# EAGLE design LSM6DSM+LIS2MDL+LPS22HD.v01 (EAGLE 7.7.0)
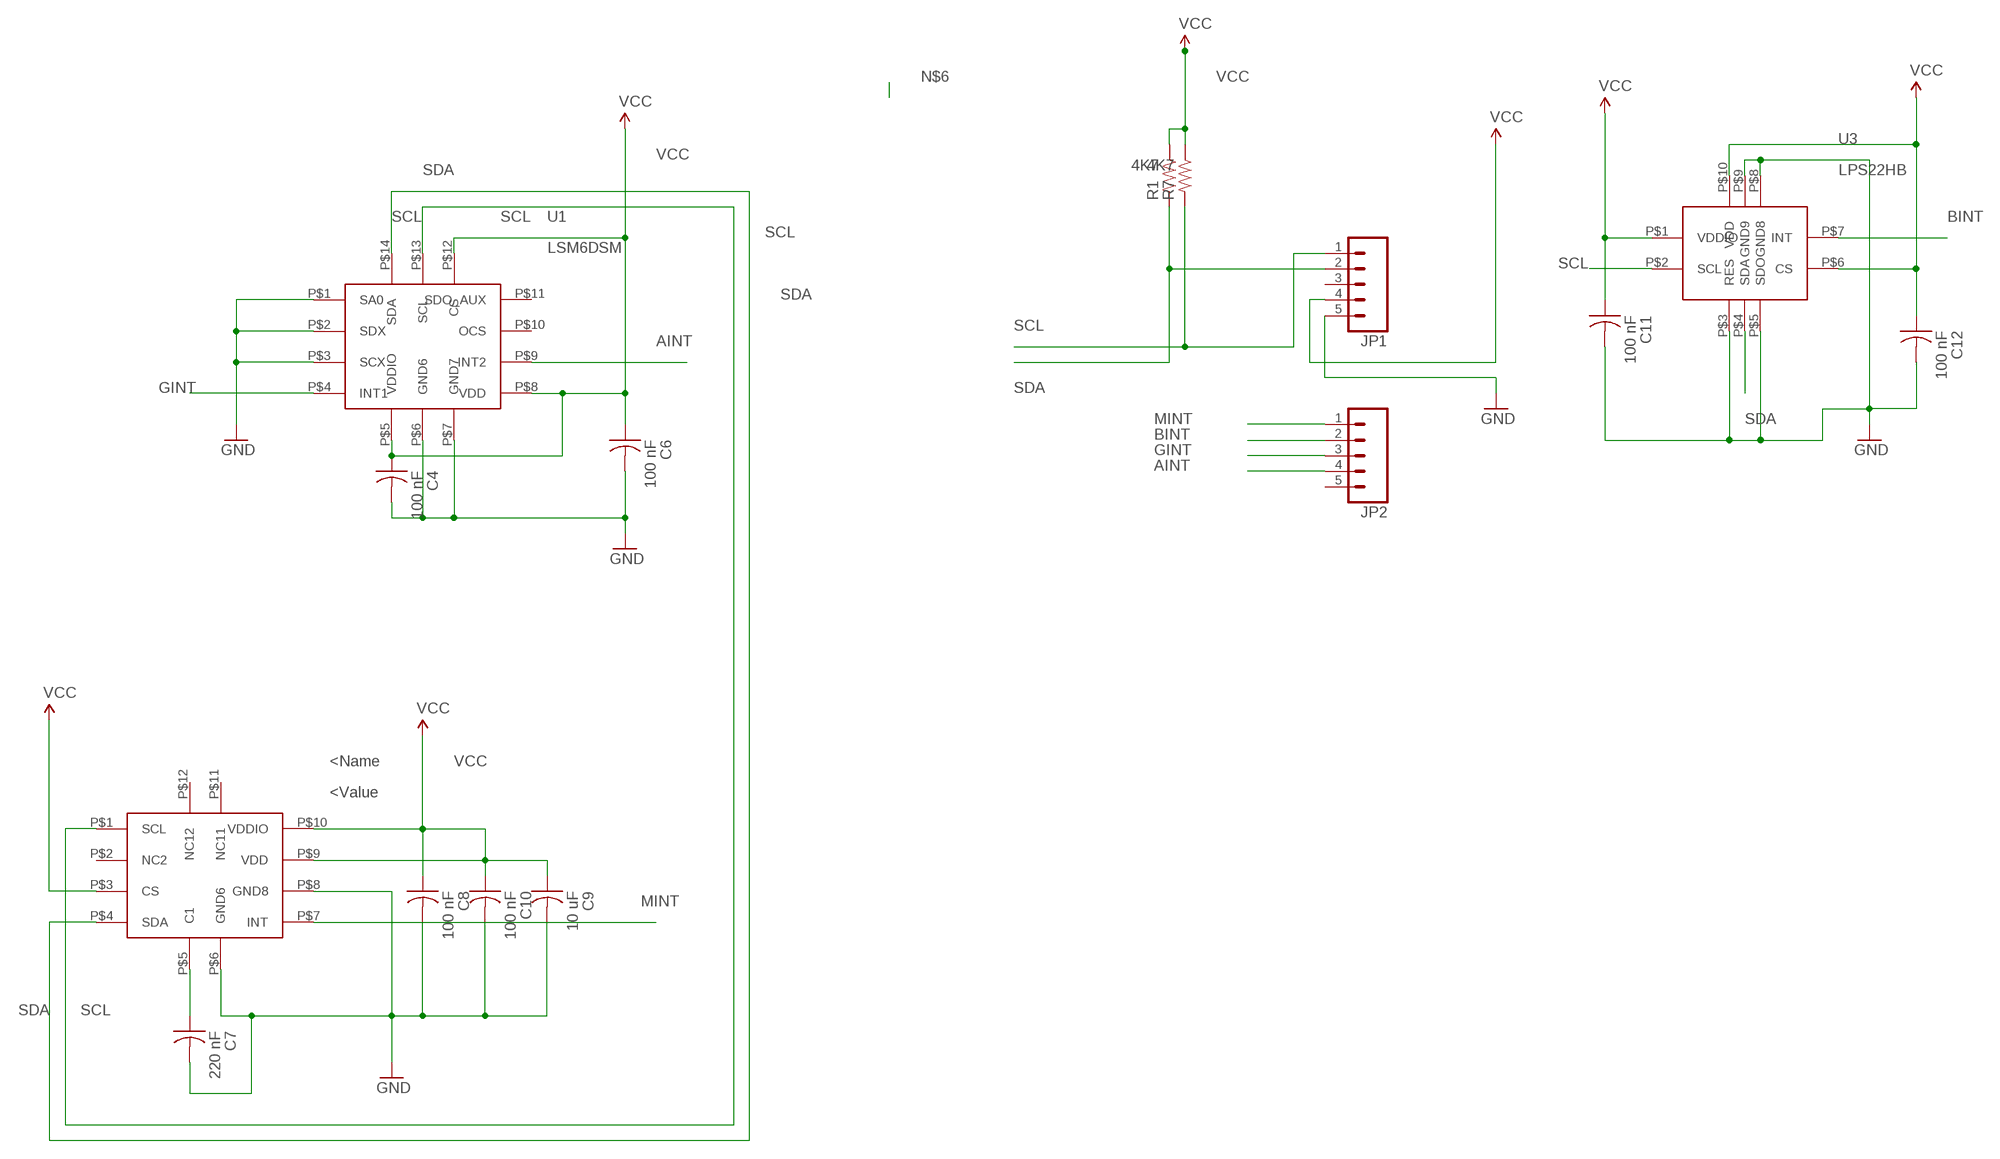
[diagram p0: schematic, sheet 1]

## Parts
C4  100 nF  C-US  [C0402_B]
C6  100 nF  C-US  [C0402_B]
C7  220 nF  C-US  [C0402_B]
C8  100 nF  C-US  [C0402_B]
C9  10 uF  C-US  [C0402_B]
C10  100 nF  C-US  [C0402_B]
C11  100 nF  C-US  [C0402_B]
C12  100 nF  C-US  [C0402_B]
JP1  M05NO_SILK  [1X05_NO_SILK]
JP2  M05NO_SILK  [1X05_NO_SILK]
R1  4K7  R-US_  [R0402_B]
R7  4K7  R-US_  [R0402_B]
U1  LSM6DSM  [LSM6DSM]
U2  LIS2MDL  [LIS2MDL]
U3  LPS22HB  [LPS22HB]

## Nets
AINT: JP2.4 U1.P$9(INT2)
BINT: JP2.2 U3.P$7(INT)
GINT: JP2.3 U1.P$4(INT1)
GND: C4.2 C6.2 C7.2 C8.2 C9.2 C10.2 C11.2 C12.2 JP1.5 U1.P$1(SA0) U1.P$2(SDX) U1.P$3(SCX) U1.P$6(GND6) U1.P$7(GND7) U2.P$6(GND6) U2.P$8(GND8) U3.P$3(RES) U3.P$5(SDO) U3.P$8(GND8) U3.P$9(GND9)
MINT: JP2.1 U2.P$7(INT)
N$4: C7.1 U2.P$5(C1)
SCL: JP1.1 R7.2 U1.P$13(SCL) U2.P$1(SCL) U3.P$2(SCL)
SDA: JP1.2 R1.2 U1.P$14(SDA) U2.P$4(SDA) U3.P$4(SDA)
VCC: C4.1 C6.1 C8.1 C9.1 C10.1 C11.1 C12.1 JP1.4 R1.1 R7.1 U1.P$5(VDDIO) U1.P$8(VDD) U1.P$12(CS) U2.P$3(CS) U2.P$9(VDD) U2.P$10(VDDIO) U3.P$1(VDDIO) U3.P$6(CS) U3.P$10(VDD)
Unconnected: JP1.3 JP2.5 U2.P$2(NC2) U2.P$11(NC11) U2.P$12(NC12)

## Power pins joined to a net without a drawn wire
OCS: U1.P$10(OCS)
SDO_AUX: U1.P$11(SDO_AUX)

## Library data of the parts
C4 C6-C12 = Spark:C-US: Capacitor
JP1 JP2 = SparkFun-Connectors:M05: Header 5 Standard 5-pin 0.1" header. Use with straight break away headers (SKU : PRT-00116), right angle break away headers (PRT-00553), swiss pins (PRT-00743), machine pins (PRT-00117), and female headers (PRT-00115). Molex polarized connector foot print use with SKU : PRT-08230 with associated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
R1 R7 = Spark:R-US_: 0402 Resistor
U1 = Kris:LSM6DSM: LSM6DSM ST accel/gyro
U2 = Kris:LIS2MDL: LIS2MDL ST magnetomneter
U3 = Kris:LPS22HB: LPS22HB ST pressure sensor http://www.st.com/content/ccc/resource/technical/document/datasheet/bf/c1/4f/23/61/17/44/8a/DM00140895.pdf/files/DM00140895.pdf/jcr:content/translations/en.DM00140895.pdf

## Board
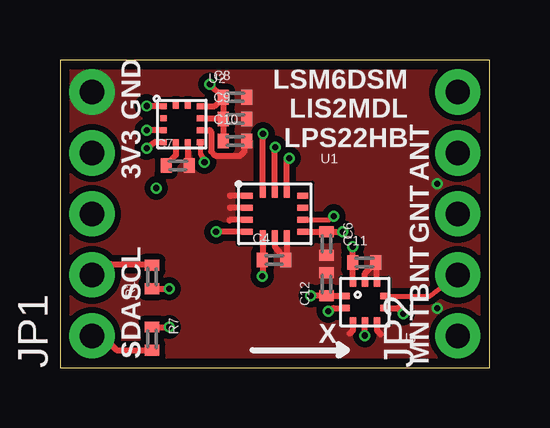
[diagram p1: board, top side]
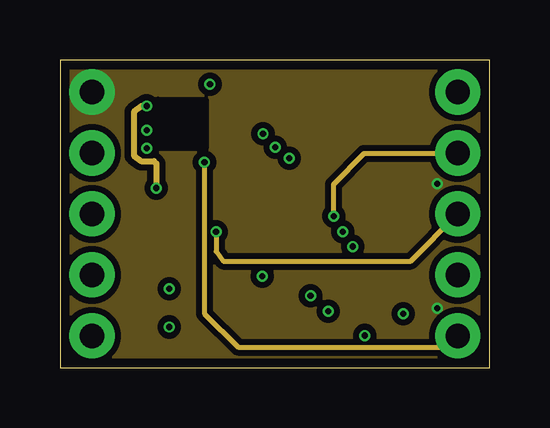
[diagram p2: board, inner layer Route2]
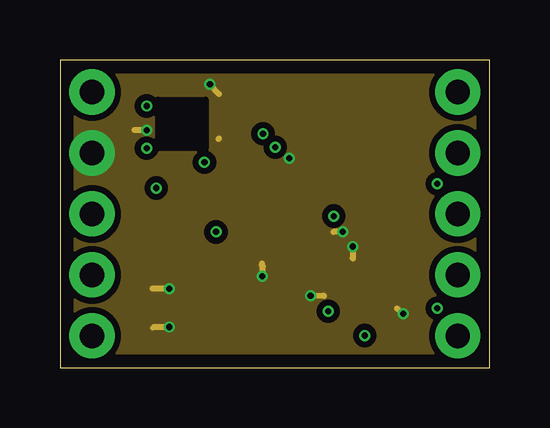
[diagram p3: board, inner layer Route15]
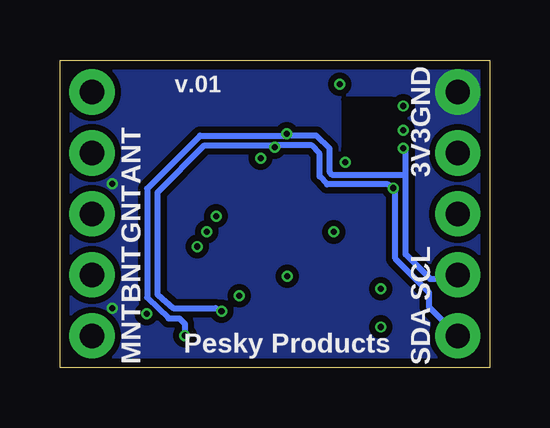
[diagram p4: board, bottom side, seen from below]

Size 17.91 x 12.83 mm. Coordinates in mm from the lower left corner, seen from the top.
Outline: 0,0 17.91,0 17.91,12.83 0,12.83 0,0
Copper layers (1*2*15*16): Top 0.035559375mm / dielectric 0.17018125mm / Route2 0.01778125mm / dielectric 47mil / Route15 0.01778125mm / dielectric 0.17018125mm / Bottom 0.035559375mm
Design rules "OSHPark-4layer *": minimum track width 5mil, minimum drill 10mil, track to track 5mil, track to pad 5mil, pad to pad 5mil, via to via 5mil, smd to smd 5mil, copper to edge 15mil, drill to drill 6mil, minimum pad ring 4mil, minimum via ring 4mil, stop-mask expansion 4mil, vias tented up to drill 20mil, thermal gap 10mil

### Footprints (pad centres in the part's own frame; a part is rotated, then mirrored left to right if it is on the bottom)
C0402_B = smd 0.457 x 0.61: 1 -0.483,0; 2 0.483,0
1X05_NO_SILK = drill 1.016 pad 1.88: 1 0,0; 2 2.54,0; 3 5.08,0; 4 7.62,0; 5 10.16,0
R0402_B = smd 0.457 x 0.61: 1 -0.483,0; 2 0.483,0
LSM6DSM = smd 0.475 x 0.25: P$1 -1.163,0.75; P$2 -1.163,0.25; P$3 -1.163,-0.25; P$4 -1.163,-0.75; P$8 1.163,-0.75; P$9 1.163,-0.25; P$10 1.163,0.25; P$11 1.163,0.75 | smd 0.25 x 0.475: P$5 -0.5,-0.912; P$6 0,-0.912; P$7 0.5,-0.912; P$12 0.5,0.912; P$13 0,0.912; P$14 -0.5,0.912
LIS2MDL = smd 0.275 x 0.25: P$1 -0.765,0.75; P$2 -0.765,0.25; P$3 -0.765,-0.25; P$4 -0.765,-0.75; P$7 0.765,-0.75; P$8 0.765,-0.25; P$9 0.765,0.25; P$10 0.765,0.75 | smd 0.25 x 0.275: P$5 -0.25,-0.765; P$6 0.25,-0.765; P$11 0.25,0.765; P$12 -0.25,0.765
LPS22HB = smd 0.3 x 0.275: P$1 -0.787,0.25; P$2 -0.787,-0.25; P$6 0.787,-0.25; P$7 0.787,0.25 | smd 0.275 x 0.3: P$3 -0.5,-0.787; P$4 0,-0.787; P$5 0.5,-0.787; P$8 0.5,0.787; P$9 0,0.787; P$10 -0.5,0.787

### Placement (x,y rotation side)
C4  8.92,4.5 0 top
C6  11.1,5.18 270 top
C7  4.9,8.43 0 top
C8  7.29,11.28 0 top
C9  7.29,10.36 0 top
C10  7.29,9.45 0 top
C11  12.67,4.39 0 top
C12  11.1,3.48 90 top
JP1  1.33,1.33 90 top
JP2  16.57,1.33 90 top
R1  3.84,3.78 90 top
R7  3.84,1.22 270 top
U1  8.95,6.41 0 top
U2  5.08,10.16 0 top
U3  12.7,2.74 0 top

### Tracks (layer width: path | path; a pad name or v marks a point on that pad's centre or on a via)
AINT  (via drill 0.25)
  Top 0.203: U1.P$9 11.22,6.16 v11.4,6.33
  Route2 0.203: v11.4,6.33 11.4,7.64 12.68,8.94 JP2.4
BINT
  Top 0.203: U3.P$7 15.41,2.99 JP2.2
GINT  (via drill 0.25)
  Top 0.254: U1.P$4 v6.5,5.66
  Route2 0.203: v6.5,5.66 6.5,4.85 6.81,4.45 14.61,4.45 JP2.3
GND  (via drill 0.25)
  Top 0.254: U1.P$3 7.08,6.16 7.06,6.15 | U1.P$2 7.1,6.66 7.09,6.68 | U1.P$1 7.11,7.16 7.09,7.19 | U1.P$6 8.95,5.04 C4.2 9.45,4.6 U1.P$7 | U3.P$9 12.7,3.94 C11.2 13.2,4.35 U3.P$8 | U3.P$5 13.2,1.56 13.36,1.4 | U3.P$3 12.2,1.56 12.06,1.42 | U2.P$6 5.33,8.66 C7.2 | U2.P$8 6.22,9.91 6.3,9.83 6.3,9.02 6.48,8.84 7.52,8.84 7.7,9.02 7.7,9.53 C10.2
  other vias: 15.72,7.67 15.72,2.49
  pour Bottom (isolate 0.254, no thermals): 0,12.83 17.91,12.83 17.91,0 10.54,0 10.39,0 0.03,0
  pour Route2 (isolate 0.254, no thermals): 0,12.83 17.91,12.83 17.91,0 10.54,0 10.39,0 0.03,0
  pour Top (isolate 0.254, no thermals): 0,12.83 17.91,12.83 17.91,0.03 0,0
MINT  (via drill 0.25)
  Top 0.203: U2.P$7 5.84,8.94 v6.02,8.56
  Route2 0.203: v6.02,8.56 6.02,2.26 7.42,0.86 16.1,0.86 JP2.1
N$1
  cutout Top (no thermals): 4.09,11.18 6.07,11.18 6.07,9.14 4.09,9.14 4.09,11.15
  cutout Route2 (no thermals): 4.09,11.18 6.07,11.18 6.07,9.14 4.09,9.14 4.09,11.15
  cutout Route15 (no thermals): 4.09,11.18 6.07,11.18 6.07,9.14 4.09,9.14 4.09,11.15
  cutout Bottom (no thermals): 4.09,11.18 6.07,11.18 6.07,9.14 4.09,9.14 4.09,11.15
N$3
  cutout Top: 11.71,3.73 13.69,3.73 13.69,1.78 11.71,1.78
N$4
  Top 0.254: U2.P$5 4.83,8.87 C7.1
N$5
  cutout Top: 7.42,7.7 10.49,7.7 10.49,5.16 7.42,5.16
SCL  (via drill 0.25)
  Top 0.254: U1.P$13 8.95,9.18 v8.97,9.2 | v11.18,2.36 11.4,2.49 U3.P$2 | U2.P$1 v3.61,10.91 | JP1.1 1.76,1.33 2.36,0.74 R7.2
  Route2 0.254: v3.61,10.91 3.39,10.91 3.07,10.67 3.07,8.84 3.38,8.61 3.91,8.61 4.01,8.51 v4.01,7.49
  Bottom 0.254: v11.18,2.36 11.43,2.49 13.18,2.49 13.84,3.05 13.84,7.32 11.89,9.27 9.07,9.27 v8.97,9.2 8.89,9.27 7.42,9.27 7.09,8.91 7.09,7.98 6.78,7.64 4.24,7.64 v4.01,7.49 3.94,7.39 3.94,4.55 2.54,3.15 2.54,2.54 JP1.1
SDA  (via drill 0.25)
  Top 0.203: 3.79,4.32 R1.2
  Top 0.254: U1.P$14 8.45,9.58 v8.46,9.75 | U2.P$4 3.95,9.41 v3.61,9.14 | v12.7,1.35 U3.P$4 | JP1.2 1.69,3.87 2.13,4.32 3.79,4.32
  Bottom 0.254: 3.5,8.05 3.5,4.72 2.49,3.71 1.5,3.71 JP1.2 | 3.5,8.05 3.5,9.02 3.52,9.07 v3.61,9.14 | v12.7,1.35 12.7,1.83 12.93,2.06 13.39,2.06 14.28,2.92 14.28,7.47 12.06,9.68 8.53,9.68 v8.46,9.75 8.26,9.68 7.24,9.68 6.68,9.14 6.68,8.18 6.58,8.05 3.5,8.05
VCC  (via drill 0.25)
  Top 0.254: v11.79,5.66 C6.1 U1.P$8 | U1.P$12 9.45,8.64 v9.55,8.74 | 8.45,4.58 8.45,3.97 v8.43,3.81 | U1.P$5 8.45,4.58 | 8.45,4.58 C4.1 | U2.P$9 6.58,10.41 C9.1 | C9.1 C10.1 | U2.P$3 3.71,9.91 v3.61,9.91 | C8.1 C9.1 | v10.44,3 C12.1 U3.P$1 | v12.19,5.05 C11.1 U3.P$10 | U3.P$6 14.07,2.49 v14.3,2.26 | C8.1 v6.25,11.81 | R7.1 v4.55,1.7 | R1.1 v4.55,3.3 | U2.P$10 6.44,10.91 C8.1
  Route15 0.203: 3.91,1.7 3.86,1.65
  Route15 0.254: v11.79,5.66 11.4,5.66 | v9.55,8.74 9.53,8.74 9.5,8.71 | v8.43,3.81 8.46,4.22 8.41,4.34 | 6.6,9.53 6.63,9.55 | v3.61,9.91 3.1,9.91 | v10.44,3 10.97,3.02 11,3 | v12.19,5.05 12.19,4.57 12.22,4.55 | v14.3,2.26 14.25,2.26 14.05,2.46 | v6.25,11.81 6.63,11.4 | v4.55,1.7 3.91,1.7 | v4.55,3.3 3.86,3.3
  pour Route15 (isolate 0.254, no thermals): 0.64,12.19 17.27,12.19 17.27,0.64 10.54,0.64 10.52,0.64 0.64,0.64

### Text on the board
tPlace: LSM6DSM / LIS2MDL / LPS22HB | GND | ANT | 3V3 | GNT | BNT | SCL | MNT | X | SDA
bPlace: GND | v.01 | 3V3 | ANT | GNT | SCL | BNT | SDA | MNT | Pesky Products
